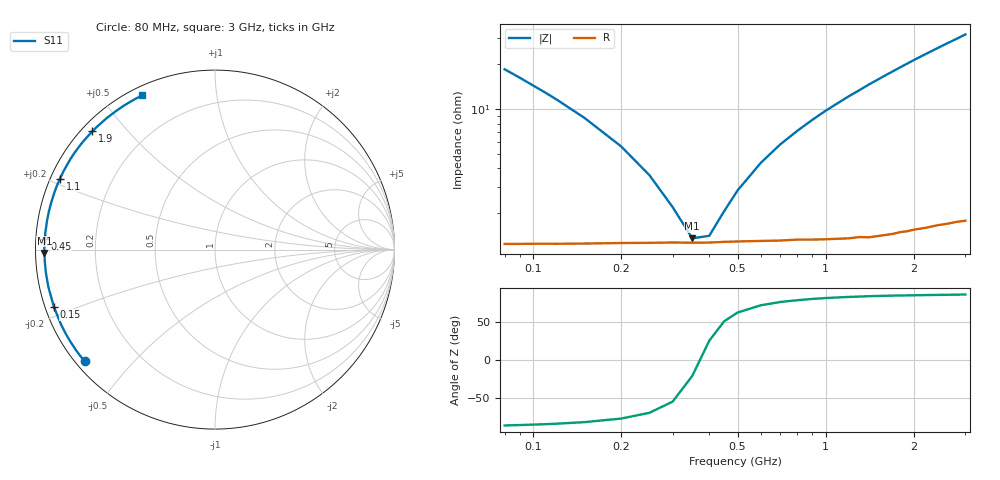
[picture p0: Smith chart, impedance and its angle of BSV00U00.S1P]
! SIEMENS Small Signal Semiconductors
! BB640
! Si Tuning Diode in SOD323
! VR = 0 V
! S-Parameters:  July  1993
# GHz  S  MA  R  50
!  f  S11
! GHz  MAG  ANG
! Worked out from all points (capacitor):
!   33 points, 80 MHz to 3 GHz, reference 50 ohm
!   read as one part to ground: C = 103 pF near 80 MHz
!   lowest |Z| = 1.35 ohm at 350 MHz (marker M1)
!   series resonance near 372 MHz, so ESL is about 1.8 nH
!   S11 on the Smith chart (normalised r, x): 80 MHz: 0.02, -0.37; 150 MHz: 0.02, -0.17; 450 MHz: 0.03, +0.03; 1.1 GHz: 0.03, +0.22; 1.9 GHz: 0.03, +0.40; 3 GHz: 0.04, +0.63
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0.08  0.9573 -139.4
0.09  0.9561 -144.0
0.1  0.9551 -147.9
0.11  0.9544 -151.1
0.12  0.9539 -153.9
0.15  0.9527 -160.4
0.2  0.9515 -167.5
0.25  0.951 -172.3
0.3  0.9506 -175.9
0.35  0.9507 -178.9
0.4  0.9506 178.6
0.45  0.9501 176.3
0.5  0.9499 174.2
0.6  0.9497 170.5
0.7  0.9497 167.1
0.9  0.9497 161.0
1  0.9499 158.1
1.1  0.95 155.4
1.2  0.9502 152.7
1.4  0.9506 147.6
1.6  0.9501 142.8
1.9  0.9494 136.0
2  0.949 133.8
2.2  0.9491 129.7
2.4  0.9489 125.8
2.6  0.9494 122.1
2.8  0.9497 118.6
3  0.9506 115.2
